TYPE AccessSDO :
STRUCT
	nIndex     	: WORD; 	(* CoE Object Index *)
    nSubIndex  	: BYTE; 	(* Subindex of CoE Object *)
	nValue		: DINT;		(* variable to be w/ r to the CoE Object *)
	bExecute	: BOOL;		(* rising edge starts w/ r to the CoE Object *)
END_STRUCT
END_TYPE
